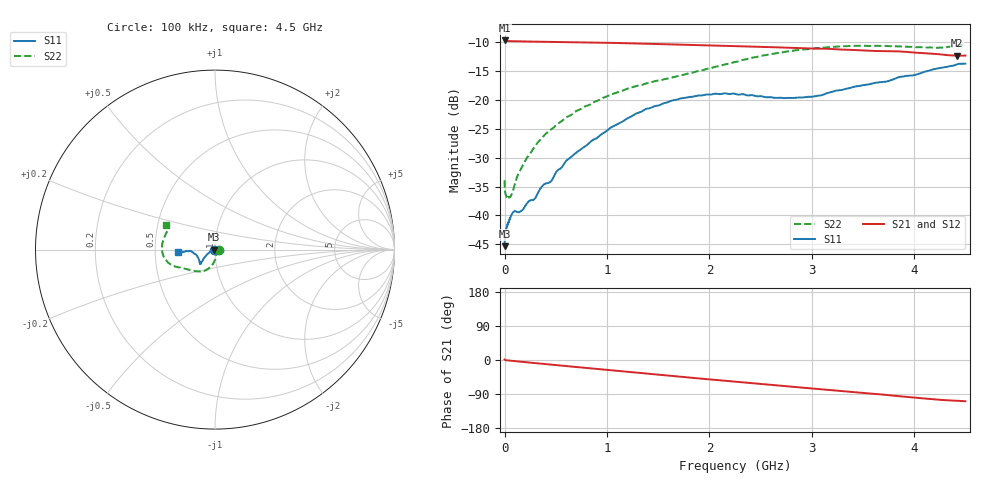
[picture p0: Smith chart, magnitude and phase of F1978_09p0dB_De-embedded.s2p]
! Integrated Device Technology
! Corporate Headquarters
! 6024 Silver Creek Valley Road
! San Jose, CA 95138  USA
! Phone:  1-408-284-8200
! Toll Free:  1-800-223-1366
! Webpage:  http://www.idt.com/
! Timing and RF Division
! 515 Groton Road, Suite 102
! Westford, MA 01886-6024
! Device:  F1978
! Description: 6-bit, 75 ohm, 0.5 dB Digital Step Attenuator
! Frequency:  5.0 MHz -  3.00 GHz
! Package:  4x4 mm QFN Plastic Package: 20 pin
! Ports:  2 RF, 11 DC
!  Pin  1  = D5 (16 dB)
!  Pin  2  = RF1  =  Port 1
!  Pin  3  = Serial Data In (DATA)
!  Pin  4  = Serial Clock (CLK)
!  Pin  5  = Serial Latch Enable (LE)
!  Pin  6  = VDD
!  Pin  7  = NC
!  Pin  8  = NC
!  Pin  9  = NC
!  Pin 10  = GND
!  Pin 11  = GND
!  Pin 12  = NC
!  Pin 13  = VMODE
!  Pin 14  = RF2  =  Port 2
!  Pin 15  = D4 (8 dB)
!  Pin 16  = D3 (4 dB)
!  Pin 17  = D2 (2 dB)
!  Pin 18  = NC
!  Pin 19  = D1 (1 dB)
!  Pin 20  = D0 (0.5 dB)
! State:  18
! Atten State:  9.0 dB
! Voltage:  +3.30 Volts
! Current:  0.592 mA
! Data:  The device was measured on a F1975 evaluation board which has
!  individual transmission lines to the RF pins.  Data was collected
!  using a calibrated network analyzer.  The evaluation board was
!  de-embedded using Automatic Fixture Removal (AFR).
!  The reference plane is the edge of the package pin.
! Misc:
!  Action Tracker AT0416
! Date Measured:  2018-02-08
! Date:  2018-03-26  MJV
! Note:
!  Integrated Device Technology supplies this data as a sample of measured
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# GHz S dB R 75
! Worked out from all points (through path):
!   291 points, 100 kHz to 4.5 GHz, reference 75 ohm
!   highest |S21| = -9.65 dB at 100 kHz (marker M1); lowest = -12.3 dB at 4.42 GHz (marker M2)
!   group delay of S21, straight-line fit = 68.5 ps
!   lowest |S11| = -45.3 dB at 100 kHz (marker M3), VSWR 1.01, Z = 74.2 + j0.0069 ohm
!   |S11| at or under -10 dB: start of sweep to end of sweep
!   |S22| runs from -36.9 to -10.3 dB; largest |S21 - S12| = 0.00017
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0.0001  -45.33 179.5  -9.65 1.2  -9.65 1.2  -33.91 -0.7
0.0006  -44.23 -176.8  -9.67 1.1  -9.67 1.1  -34.79 -3.7
0.002  -43.32 -174.7  -9.70 0.8  -9.69 0.8  -35.51 -4.6
0.02  -42.04 -173.4  -9.73 -0.8  -9.73 -0.8  -36.77 -21.2
0.055  -40.41 -169.7  -9.76 -1.8  -9.76 -1.8  -36.79 -41.5
0.08  -39.48 -164.1  -9.78 -2.4  -9.78 -2.4  -35.83 -55.6
0.14  -39.46 -158.0  -9.80 -4.0  -9.80 -4.0  -32.58 -68.3
0.32  -36.29 -162.7  -9.86 -8.8  -9.86 -8.8  -27.42 -84.0
0.38  -34.68 -157.9  -9.88 -10.3  -9.88 -10.3  -26.25 -86.0
0.46  -33.95 -159.6  -9.90 -12.4  -9.90 -12.4  -24.99 -89.5
0.6  -30.55 -157.2  -9.94 -15.9  -9.94 -15.9  -23.02 -94.7
0.76  -28.33 -151.7  -9.98 -20.0  -9.98 -20.0  -21.36 -100.1
1.04  -24.72 -146.8  -10.07 -27.3  -10.07 -27.3  -19.05 -108.9
1.38  -21.53 -141.3  -10.22 -35.9  -10.22 -35.9  -17.11 -120.6
1.52  -20.82 -138.8  -10.26 -39.3  -10.26 -39.3  -16.57 -125.3
1.88  -19.24 -135.7  -10.46 -48.2  -10.45 -48.2  -15.00 -139.5
2.26  -18.95 -137.8  -10.64 -57.4  -10.63 -57.4  -13.34 -151.7
2.64  -19.61 -149.2  -10.83 -66.5  -10.83 -66.5  -11.91 -160.0
3.02  -19.36 -164.2  -11.05 -75.5  -11.04 -75.5  -11.04 -168.4
3.76  -16.62 -176.5  -11.50 -92.8  -11.49 -92.8  -10.63 171.4
4.42  -13.78 -175.1  -12.30 -107.6  -12.29 -107.6  -10.52 155.0
4.5  -13.67 -177.0  -12.26 -108.8  -12.26 -108.8  -10.26 153.6
